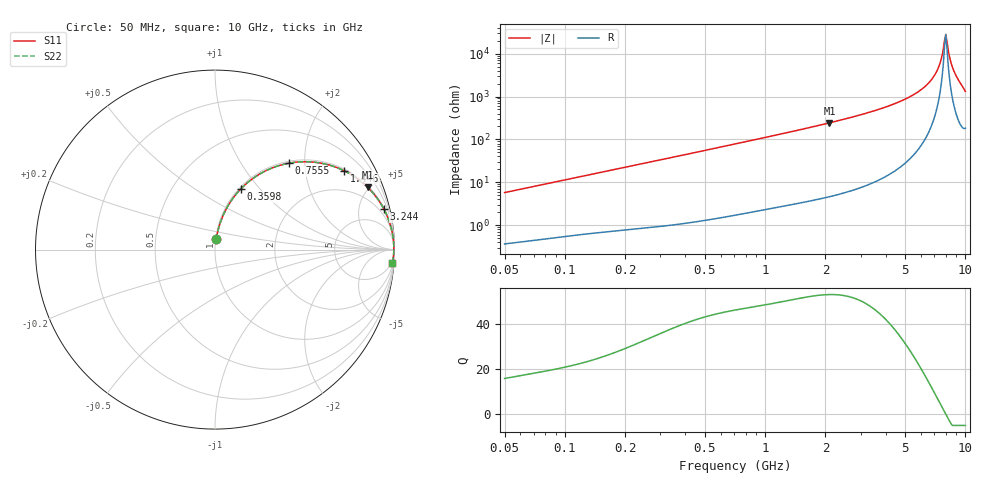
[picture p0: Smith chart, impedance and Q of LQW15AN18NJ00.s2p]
!Murata Part Number: LQW15AN18NJ00
!These Parameters are Measured in Series Mode Connection
!  o--[Z]--o
!Port1  Port2
!  o-------o
!Freq. Start=50[MHz] Stop=10[GHz], 401[Steps]
# Hz S RI R 50
!Freq.(Hz)	S 11(Real)	S 11(Imag)	S 21(Real)	S 21(Imag)	S 12(Real)	S 12(Imag)	S 22(Real)	S 22(Imag)
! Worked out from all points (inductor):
!   401 points, 50 MHz to 10 GHz, reference 50 ohm
!   read as one part in series: L = 18.1 nH near 51.34 MHz
!   highest Q = 52.8 at 2.095 GHz (marker M1), where L = 18.4 nH
!   self-resonance near 7.879 GHz
!   S11 on the Smith chart (normalised r, x): 50 MHz: 1.01, +0.11; 359.8 MHz: 1.02, +0.80; 755.5 MHz: 1.04, +1.67; 1.446 GHz: 1.06, +3.24; 3.244 GHz: 1.17, +8.32; 10 GHz: 5, -26
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5e7  0.00686 0.0567  0.9931 -0.0567  0.9931 -0.0567  0.00686 0.0567
1.214486e8  0.0239 0.1323  0.9761 -0.1323  0.9761 -0.1323  0.0239 0.1323
2.949953e8  0.103 0.2901  0.897 -0.2901  0.897 -0.2901  0.103 0.2901
3.598352e8  0.1429 0.3373  0.8571 -0.3373  0.8571 -0.3373  0.1429 0.3373
7.071068e8  0.3811 0.4749  0.6189 -0.4749  0.6189 -0.4749  0.3811 0.4749
7.555233e8  0.4122 0.4816  0.5878 -0.4816  0.5878 -0.4816  0.4122 0.4816
1.445853e9  0.7207 0.439  0.2793 -0.439  0.2793 -0.439  0.7207 0.439
1.717543e9  0.7872 0.3998  0.2128 -0.3998  0.2128 -0.3998  0.7872 0.3998
2.095058e9  0.8504 0.3474  0.1496 -0.3474  0.1496 -0.3474  0.8504 0.3474
3.243629e9  0.9412 0.2251  0.0588 -0.2251  0.0588 -0.2251  0.9412 0.2251
4.171863e9  0.9701 0.1583  0.0299 -0.1583  0.0299 -0.1583  0.9701 0.1583
5.509778e9  0.9884 0.0893  0.0116 -0.0893  0.0116 -0.0893  0.9884 0.0893
6.632392e9  0.9946 0.0449  0.00543 -0.0449  0.00543 -0.0449  0.9946 0.0449
7.276762e9  0.9961 0.0227  0.00393 -0.0227  0.00393 -0.0227  0.9961 0.0227
7.571744e9  0.9964 0.013  0.00362 -0.013  0.00362 -0.013  0.9964 0.013
7.775012e9  0.9965 0.00639  0.00354 -0.00639  0.00354 -0.00639  0.9965 0.00639
7.983737e9  0.9964 -0.000257  0.00355 0.000257  0.00355 0.000257  0.9964 -0.000257
8.090191e9  0.9964 -0.00363  0.0036 0.00363  0.0036 0.00363  0.9964 -0.00363
8.418147e9  0.9961 -0.014  0.00393 0.014  0.00393 0.014  0.9961 -0.014
8.759398e9  0.9954 -0.0248  0.0046 0.0248  0.0046 0.0248  0.9954 -0.0248
9.236013e9  0.9936 -0.0406  0.00635 0.0406  0.00635 0.0406  0.9936 -0.0406
1e10  0.984 -0.0736  0.016 0.0736  0.016 0.0736  0.984 -0.0736
